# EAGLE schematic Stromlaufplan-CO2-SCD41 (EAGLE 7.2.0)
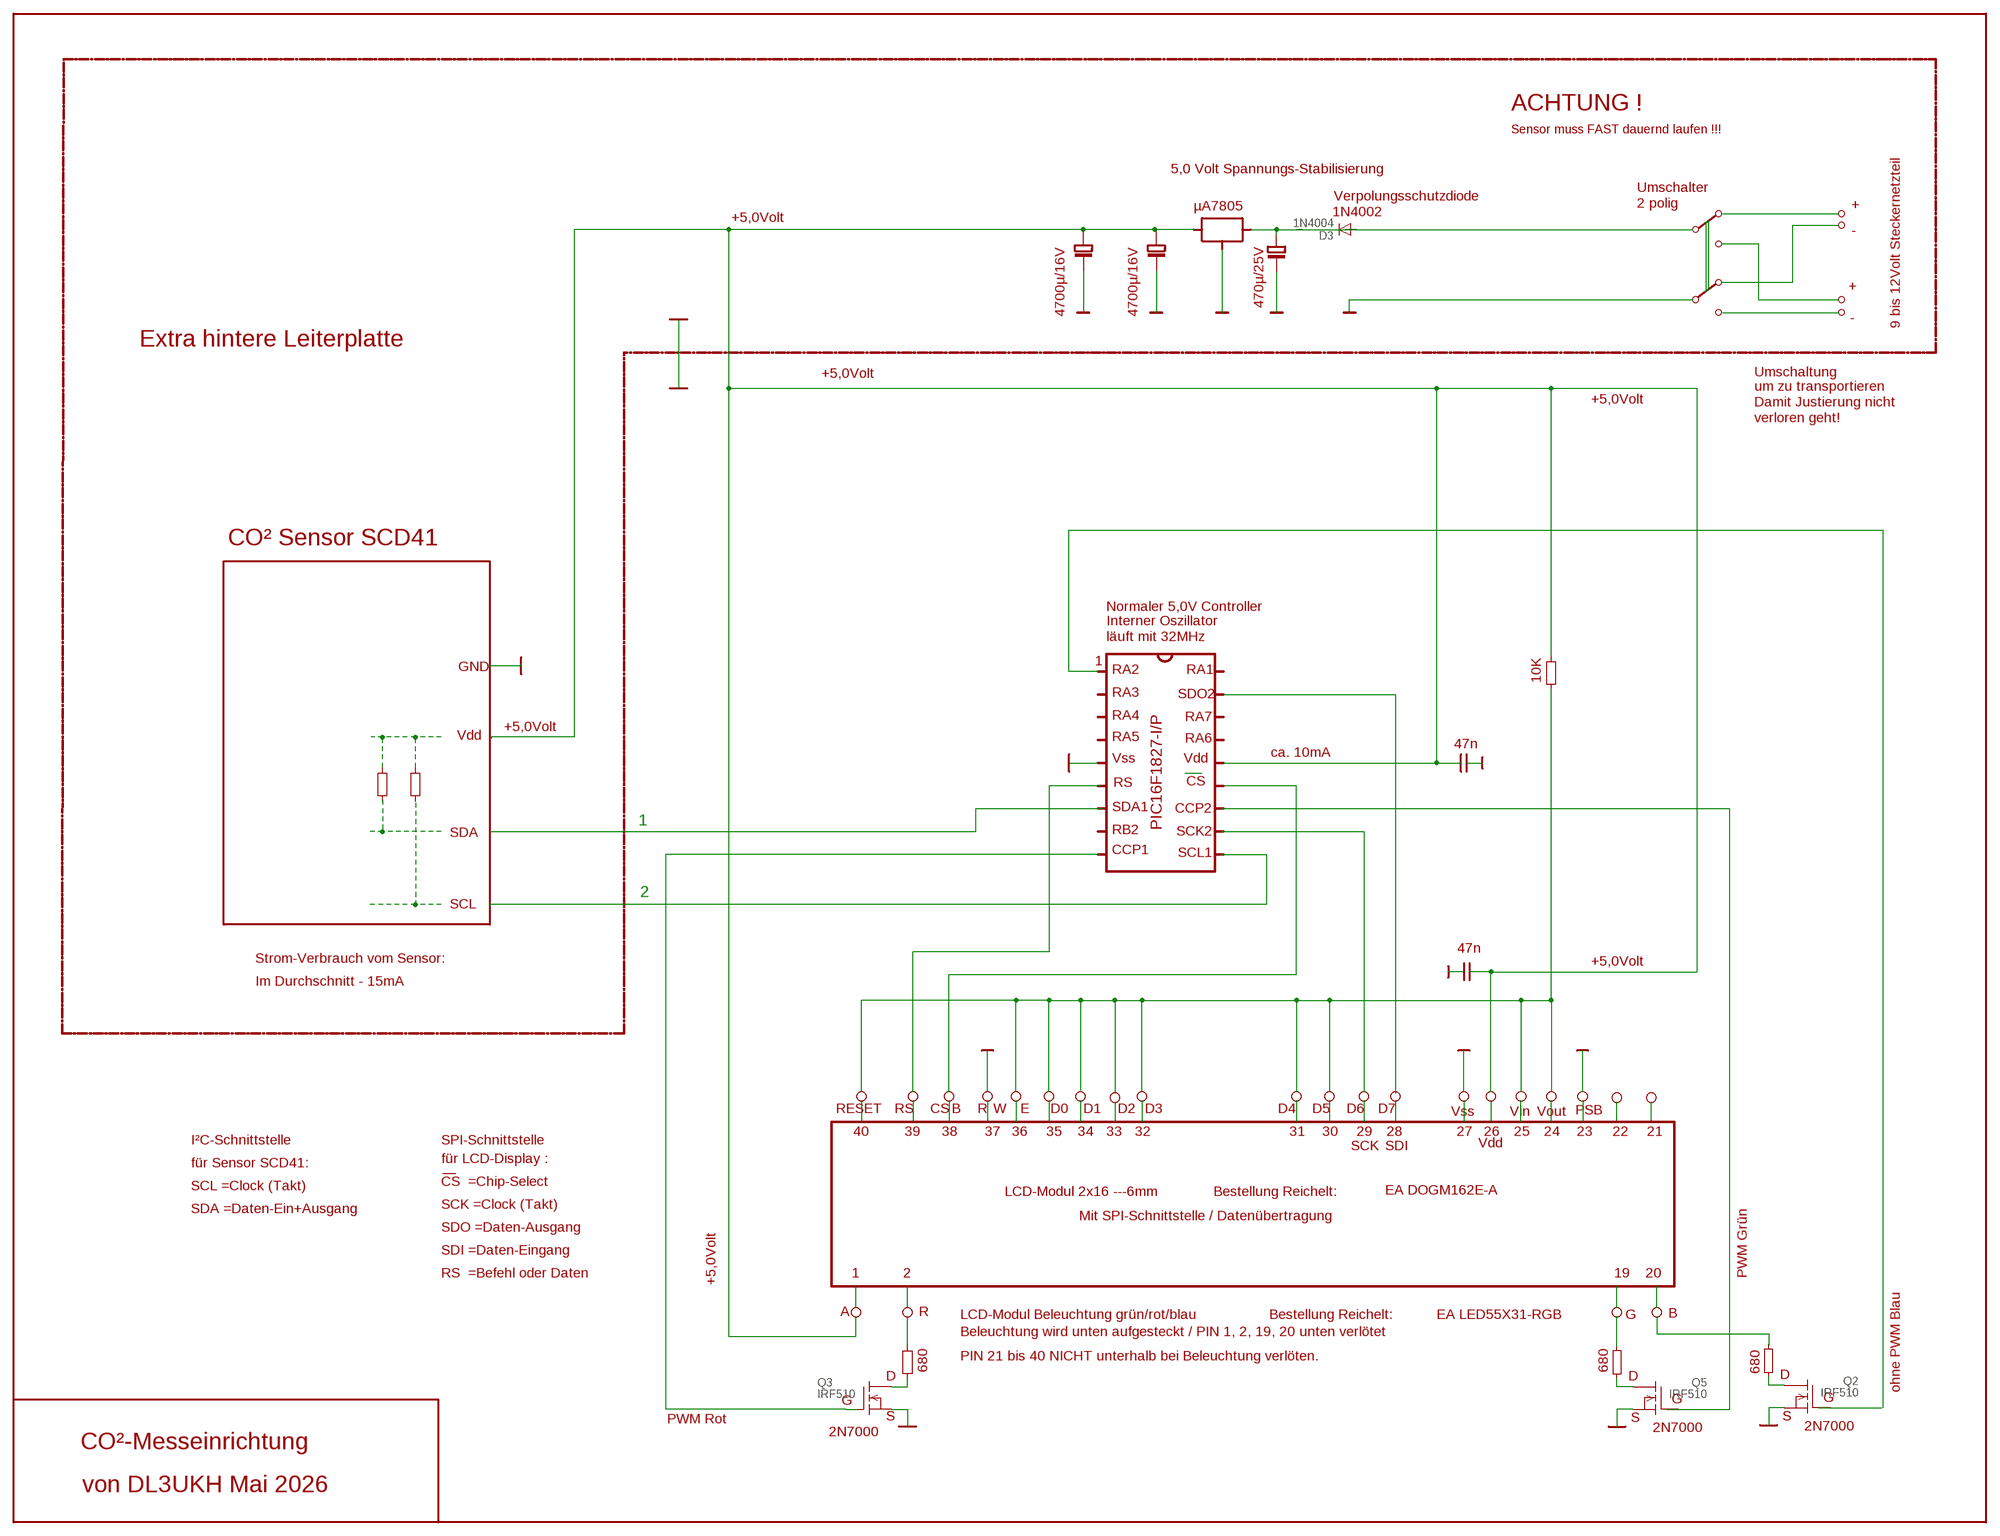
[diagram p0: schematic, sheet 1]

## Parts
D3  1N4004  [DO41-10]
Q2  IRF510  [TO220]
Q3  IRF510  [TO220]
Q5  IRF510  [TO220]

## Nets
N$47: D3.C
N$56: Q3.2(D)
N$58: Q3.3(S)
N$59: Q3.1(G)
N$60: Q5.1(G)
N$61: Q5.2(D)
N$63: Q5.3(S)
N$64: Q2.2(D)
N$87: D3.A
N$96: Q2.3(S)
N$97: Q2.1(G)

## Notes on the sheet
- ACHTUNG !
- Sensor muss FAST dauernd laufen !!!
- 5,0 Volt Spannungs-Stabilisierung
- Umschalter
- Verpolungsschutzdiode
- µA7805 | 2 polig | +
- 1N4002
- +5,0Volt
- -
- +
- 470µ/25V
- 4700µ/16V | 4700µ/16V
- -
- 9 bis 12Volt Steckernetzteil
- Extra hintere Leiterplatte
- +5,0Volt | Umschaltung
- um zu transportieren
- +5,0Volt | Damit Justierung nicht
- verloren geht!
- CO² Sensor SCD41
- Normaler 5,0V Controller
- Interner Oszillator
- läuft mit 32MHz
- 1
- GND | RA2 | RA1
- 10K
- RA3 | SDO2
- RA4 | RA7
- +5,0Volt
- Vdd | RA5 | RA6
- 47n
- ca. 10mA
- Vss | Vdd
- RS | CS
- SDA1 | CCP2
- 1 | PIC16F1827-I/P
- SDA | RB2 | SCK2
- CCP1 | SCL1
- 2
- SCL
- 47n
- Strom-Verbrauch vom Sensor: | +5,0Volt
- Im Durchschnitt - 15mA
- RESET | RS | CS | B | R | W | E | D0 | D1 | D2 | D3 | D4 | D5 | D6 | D7 | Vss | Vin | Vout | PSB
- 40 | 39 | 38 | 37 | 36 | 35 | 34 | 33 | 32 | 31 | 30 | 29 | 28 | 27 | 26 | 25 | 24 | 23 | 22 | 21
- I²C-Schnittstelle | SPI-Schnittstelle | Vdd
- SCK | SDI
- für LCD-Display :
- für Sensor SCD41:
- CS  =Chip-Select
- SCL =Clock (Takt)
- LCD-Modul 2x16 ---6mm | Bestellung Reichelt: | EA DOGM162E-A
- SCK =Clock (Takt)
- SDA =Daten-Ein+Ausgang
- Mit SPI-Schnittstelle / Datenübertragung
- SDO =Daten-Ausgang
- SDI =Daten-Eingang
- RS  =Befehl oder Daten | 1 | 2 | 19 | 20 | PWM Grün
- +5,0Volt
- A | R | LCD-Modul Beleuchtung grün/rot/blau | Bestellung Reichelt: | EA LED55X31-RGB | G | B
- Beleuchtung wird unten aufgesteckt / PIN 1, 2, 19, 20 unten verlötet
- PIN 21 bis 40 NICHT unterhalb bei Beleuchtung verlöten.
- 680 | 680 | 680
- D | D | D
- ohne PWM Blau
- G | G | G
- PWM Rot | S | S | S
- 2N7000 | 2N7000
- 2N7000
- CO²-Messeinrichtung
- von DL3UKH Mai 2026

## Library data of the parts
D3 = diode:1N4004: DIODE
Q2 Q3 Q5 = transistor-fet:IRF510: N-Channel Enhancement MOSFET (HEXFET); 100V; 5,6A; 0,54Ohm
